FUNCTION_BLOCK FB96
TITLE =Get Quick Stop State
//*****************************************************************************
//* maxon motor ag
//* R&D
//* all rights reserved
//*****************************************************************************
//* Summary:  Read device status
//*
//* Remarks:
//*
//* Created under: STEP7 REV5.2+SP1
//*****************************************************************************
//* History:
//* 19.05.2004 | INA   first release
//*
//*
//*****************************************************************************
//

AUTHOR:INA
FAMILY:StateMac
NAME:GetQuick
VERSION:00.01


VAR_INPUT

Read : BOOL //A rising edge start the command

  NodeID : BYTE //Adress of the maxon device

END_VAR
VAR_OUTPUT
  Done : BOOL //Data valid flag is TRUE if data were available

  Err : BOOL //Error flag is TRUE if an Error has occured, see ErrNo for more details

  ErrNo : DINT //Contains detailed error information

  IsStopped : BOOL //Device quick stop state

END_VAR
VAR
  xEdgeMerker : BOOL //Edge Merker

  xEdgeFlag : BOOL //Edge Flag

  xStep : INT
  xStatusword : WORD
  xQuickStopActiv : WORD  := W#16#7
END_VAR

BEGIN

NETWORK
TITLE = Activate the service function
//

// SDO Read "Get Quick Stop State"

       U    #Read
       FP   #xEdgeFlag                   // recognize a positiv edge of the Read signal
       =    #xEdgeMerker                 // and set the xEdgeMerker for one cycle to true

       L    #xStep
       L    0
       ==I
       U    #xEdgeMerker
       SPB  nstp                         // iStep = 1 -> fnc1

       L    #xStep                       // jump list
       SPL  List
       SPA  rdef
       SPA  fnc1
       SPA  fncE
List  :SPA  rdef

rdef  :NOP  0
       R    #Done                        // reset Done
       R    #Err                         // reset Error
       L    0
       T    #xStep                       // iStep = 0
       SPA  end

fnc1  :NOP  0
       CALL FC1
         NodeID:=#NodeID
         Index:=DW#16#00006041
         SubIndex:=DW#16#00000000
         RET_VAL:=#Done
         Err:=#Err
         ErrNo:=#ErrNo

       L    DB219.DBW10
       UW   W#16#006F
       T    #xStatusword

       L    #xStatusword
       L    #xQuickStopActiv
       ==I
       SPB  tdis
       SPA  fdis

tdis  :NOP  0
       S    #IsStopped                   // set IsStopped
       SPA  fncE

fdis  :NOP  0
       R    #IsStopped                   // reset IsStopped

fncE  :NOP  0
       L    0
       T    #xStep
       SPA  end

nstp  :NOP  0
       L    #xStep
       INC            1
       T    #xStep

end   :NOP  0
END_FUNCTION_BLOCK
